FUNCTION F_Crc4 : BYTE
VAR_INPUT
END_VAR
VAR_IN_OUT
	aData			: ARRAY[*] OF USINT;
END_VAR
VAR
	nLowBoundData	: DINT;			// lower index
	nUpBoundData	: DINT;
	nIdxCntData		: DINT;
	
	aCrcTable 		: ARRAY[0..15] OF BYTE:=[ 0,13,7,10,14,3,9,4,1,12,6,11,15,2,8,5];		// CRC lookup table
	nIdx			: DINT;
	nRetBuff		: BYTE;
END_VAR

// check if input array is not there
IF aData <> 0 THEN
	// get array dimensions 
	nLowBoundData := LOWER_BOUND(aData, 1);
	nUpBoundData := UPPER_BOUND(aData, 1);
	IF nLowBoundData = nUpBoundData THEN
		nIdxCntData := 1;
	ELSE
		nIdxCntData := nUpBoundData - nLowBoundData + 1;	
	END_IF


	nRetBuff:=5;
	
	FOR nIdx := nLowBoundData TO nUpBoundData DO
		nRetBuff := aData[nIdx] XOR aCrcTable[nRetBuff];
	END_FOR
	
	nRetBuff := 0 XOR aCrcTable[nRetBuff];

END_IF

 F_Crc4 := nRetBuff;

END_FUNCTION
